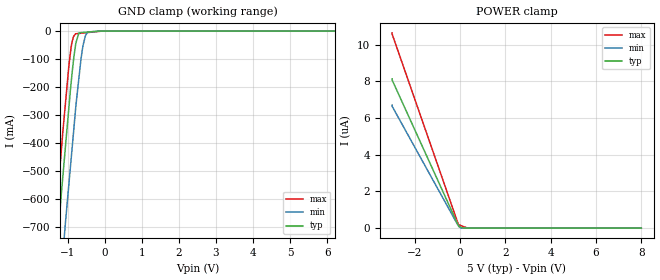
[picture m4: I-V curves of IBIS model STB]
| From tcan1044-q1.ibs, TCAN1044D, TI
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|   STB Model
[Model]   STB
Model_type   Input
Vinl = 1.5
Vinh = 3.5
|   typ   min   max
C_comp   5.708e-12   5.416e-12   5.769e-12
[Voltage Range]   5   4.5   5.5
[Temperature Range]   25   150   -55
[Power Clamp Reference]   5   4.5   5.5
[GND Clamp Reference]   0   0   0
[GND Clamp]
|   Voltage   I(typ)   I(min)   I(max)
-3V       -3.691A    -3.919A    -3.582A
-1.522V   -1.152A    -1.424A    -1.002A
-1.335V   -840.5mA   -1.117A    -686.6mA
-1.302V   -786.7mA   -1.064A    -630.7mA
-1.17V    -572.4mA   -853.8mA   -416.5mA
-1.055V   -398.2mA   -669.7mA   -243.5mA
-917mV    -191.1mA   -465.7mA   -62.73mA
-793.3mV  -51.22mA   -282.6mA   -9.674mA
-702.7mV  -6.375mA   -169.3mA   -8.463mA
-607.6mV  -5.219mA   -65.45mA   -7.192mA
-461mV    -3.438mA   -3.797mA   -5.232mA
8V        0A         0A         0A
[POWER Clamp]
|   Voltage   I(typ)   I(min)   I(max)
-3V       8.144uA    6.709uA    10.65uA
-3V       8.086uA    6.652uA    10.59uA
-123.7mV  274.1nA    229.6nA    378nA
-71.1mV   131.2nA    159.1nA    191.2nA
-51.9mV   79.05nA    133.3nA    182.2nA
47.48mV   47.8nA     0A         135.4nA
335.2mV   0A         0A         0A
8V        0A         0A         0A
